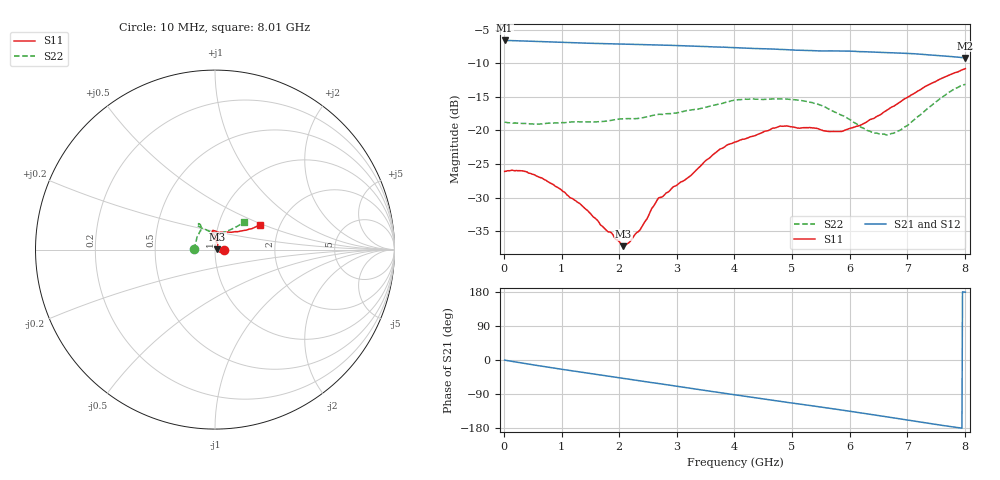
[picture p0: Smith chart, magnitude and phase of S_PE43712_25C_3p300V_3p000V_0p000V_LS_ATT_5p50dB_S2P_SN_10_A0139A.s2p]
! DEVICE ID: PE43712
! File Path: z:\PE43713\PE43713_CHAR_NOM_04292014\AMB\3p300\LS_ATT_5p50dB\PE43713_AMB_3p300V_3p000V_0p000V_LS_ATT_5p50dB_S2P_SN_10_A0139A.s2p
! Serial: 10
! Lot: A0139A
! Temp: 25C
! VDD: 3.300
! VSS: 0.000
! Control_Hi: 3.000
! Control_Lo: 0.000
! Attenuation Step: 5.50dB
! Port 1: RF1
! Port 2: RF2
! ThroughPath:1-2
! IDD: 0.0001472175
! ISS: -1.619e-007
#  Hz  S  RI  R  50
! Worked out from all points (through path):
!   801 points, 10 MHz to 8.01 GHz, reference 50 ohm
!   highest |S21| = -6.61 dB at 10 MHz (marker M1); lowest = -9.2 dB at 8.01 GHz (marker M2)
!   group delay of S21, straight-line fit = 62.1 ps
!   lowest |S11| = -37.2 dB at 2.07 GHz (marker M3), VSWR 1.03, Z = 51.4 + j0.214 ohm
!   |S11| at or under -10 dB: start of sweep to end of sweep
!   |S22| runs from -20.7 to -13.1 dB; largest |S21 - S12| = 0.0015
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1e7  0.0495 -0.0001  0.4675 -0.00268  0.4673 -0.00247  -0.1153 0.000673
3.4e8  0.0488 -0.0096  0.4576 -0.0703  0.4574 -0.0692  -0.1121 0.00962
6.3e8  0.0422 -0.0142  0.4415 -0.1245  0.4415 -0.1245  -0.1102 0.0181
9.6e8  0.0334 -0.0156  0.4155 -0.1807  0.4157 -0.1807  -0.1105 0.0281
1.35e9  0.0242 -0.0133  0.3781 -0.2389  0.3781 -0.2389  -0.1085 0.0404
2.07e9  0.0136 0.00208  0.2914 -0.3285  0.2915 -0.3284  -0.1005 0.0694
2.17e9  0.0138 0.00477  0.2777 -0.3388  0.2777 -0.3387  -0.0983 0.073
2.36e9  0.0135 0.0121  0.25 -0.357  0.25 -0.3569  -0.092 0.082
2.68e9  0.016 0.0269  0.2022 -0.381  0.2022 -0.3811  -0.0824 0.1029
3.23e9  0.00815 0.0449  0.1133 -0.4095  0.1134 -0.4096  -0.0786 0.1177
3.72e9  0.00312 0.0709  0.0336 -0.4162  0.0333 -0.4162  -0.08 0.1349
4.01e9  -0.00334 0.0818  -0.0136 -0.4131  -0.0137 -0.4131  -0.0881 0.1431
4.79e9  -0.013 0.1068  -0.1303 -0.3794  -0.1303 -0.3797  -0.0971 0.1421
5.35e9  -0.00176 0.1044  -0.2017 -0.3371  -0.2016 -0.3368  -0.0934 0.1314
5.63e9  0.0111 0.0975  -0.2338 -0.313  -0.2337 -0.3132  -0.0775 0.1222
5.87e9  0.0251 0.0952  -0.2624 -0.2887  -0.2619 -0.2887  -0.0598 0.1145
6.39e9  0.0726 0.0975  -0.3104 -0.2253  -0.3098 -0.225  -0.0138 0.0956
6.68e9  0.106 0.0984  -0.3309 -0.1849  -0.3304 -0.1849  0.017 0.0914
6.99e9  0.1412 0.1031  -0.3474 -0.1398  -0.3469 -0.1398  0.0484 0.0965
7.35e9  0.1848 0.1124  -0.3557 -0.0851  -0.3554 -0.085  0.0905 0.1135
7.73e9  0.2255 0.1259  -0.354 -0.0297  -0.3539 -0.0299  0.1357 0.137
8.01e9  0.252 0.1396  -0.347 0.00621  -0.3463 0.00556  0.1591 0.1523
